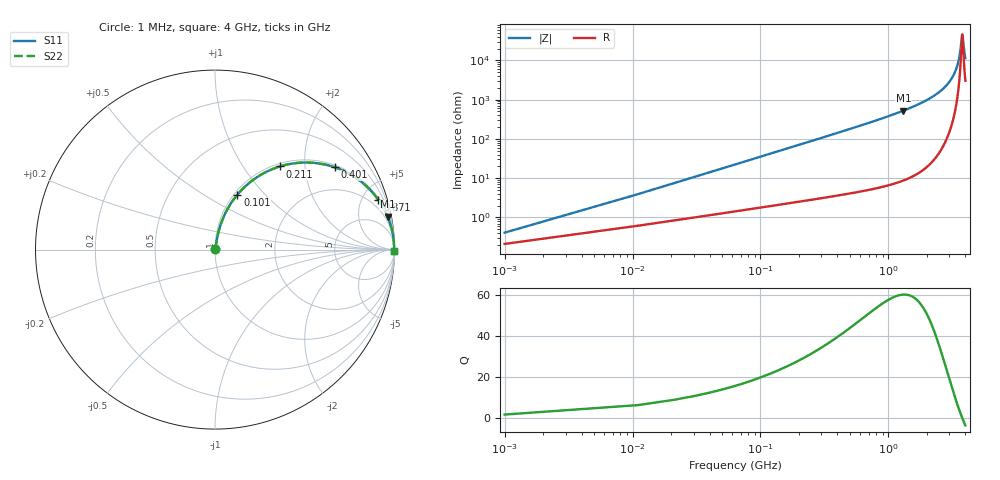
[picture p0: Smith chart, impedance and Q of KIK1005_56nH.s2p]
!version-3
!date-01.2023
!Series
# MHz S RI R 50
!Freq ReS11 ImS11 ReS21 ImS21 ReS12 ImS12 ReS22 ImS22
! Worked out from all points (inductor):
!   401 points, 1 MHz to 4 GHz, reference 50 ohm
!   read as one part in series: L = 56 nH near 21 MHz
!   highest Q = 60.1 at 1.311 GHz (marker M1), where L = 63.7 nH
!   self-resonance near 3.771 GHz
!   S11 on the Smith chart (normalised r, x): 1 MHz: 1.00, +0.01; 101 MHz: 1.04, +0.71; 211 MHz: 1.05, +1.49; 401 MHz: 1.07, +2.85; 871 MHz: 1.12, +6.47; 4 GHz: open
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1  0.00213 0.0035  0.9979 -0.0035  0.9979 -0.0035  0.00213 0.0035
31  0.0214 0.1057  0.9786 -0.1057  0.9786 -0.1057  0.0214 0.1057
41  0.0311 0.1382  0.9689 -0.1382  0.9689 -0.1382  0.0311 0.1382
61  0.0561 0.1998  0.9439 -0.1998  0.9439 -0.1998  0.0561 0.1998
101  0.1245 0.3059  0.8755 -0.3059  0.8755 -0.3059  0.1245 0.3059
151  0.2302 0.4009  0.7698 -0.4009  0.7698 -0.4009  0.2302 0.4009
211  0.3616 0.4634  0.6384 -0.4634  0.6384 -0.4634  0.3616 0.4634
401  0.6668 0.4588  0.3332 -0.4588  0.3332 -0.4588  0.6668 0.4588
671  0.8511 0.3461  0.1489 -0.3461  0.1489 -0.3461  0.8511 0.3461
871  0.9087 0.2791  0.0913 -0.2791  0.0913 -0.2791  0.9087 0.2791
1311  0.9621 0.1829  0.0379 -0.1829  0.0379 -0.1829  0.9621 0.1829
1341  0.9641 0.178  0.0359 -0.178  0.0359 -0.178  0.9641 0.178
2001  0.9877 0.1008  0.0123 -0.1008  0.0123 -0.1008  0.9877 0.1008
2671  0.9954 0.0529  0.00463 -0.0529  0.00463 -0.0529  0.9954 0.0529
3061  0.9971 0.0318  0.00289 -0.0318  0.00289 -0.0318  0.9971 0.0318
3341  0.9977 0.0185  0.00231 -0.0185  0.00231 -0.0185  0.9977 0.0185
3581  0.9979 0.00812  0.00214 -0.00812  0.00214 -0.00812  0.9979 0.00812
3651  0.9979 0.00522  0.00214 -0.00522  0.00214 -0.00522  0.9979 0.00522
3771  0.9978 0.000379  0.00218 -0.000379  0.00218 -0.000379  0.9978 0.000379
3801  0.9978 -0.000806  0.0022 0.000806  0.0022 0.000806  0.9978 -0.000806
3911  0.9977 -0.00507  0.0023 0.00507  0.0023 0.00507  0.9977 -0.00507
4000  0.9976 -0.00844  0.0024 0.00844  0.0024 0.00844  0.9976 -0.00844
